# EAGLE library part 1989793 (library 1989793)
PCB terminal block, nominal current: 2 A, rated voltage (III/2): 250 V, nominal cross section: 0.5 mm, number of potentials: 7, number of rows: 1, number of positions per row: 7, product range: PTSA 0,5, pitch: 2.5 mm, connection method: Push-in spring connection, mounting: Wave soldering, conductor/PCB connection direction: 45 , color: green, Pin layout: Linear pinning, Solder pin [P]: 3.6 mm, number of solder pins per potential: 1, type of packaging: packed in cardboard. Soldering legs in front area, on Source: Datasheet
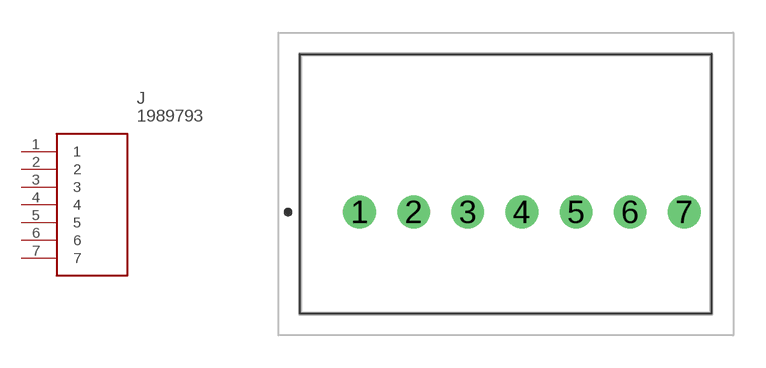
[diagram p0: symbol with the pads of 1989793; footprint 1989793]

Designator prefix J

## 1989793 (Description: PCB terminal block, nominal current: 2 A, rated voltage (III/2): 250 V, nominal cross section: 0.5 mm, number of potentials: 7, number of rows: 1, number of positions per row: 7, product range: PTSA 0,5, pitch: 2.5 mm, connection method: Push-in spring connection, mounting: Wave soldering, conductor/PCB connection direction: 45 , color: green, Pin layout: Linear pinning, Solder pin [P]: 3.6 mm, number of solder pins per potential: 1, type of packaging: packed in cardboard. Soldering legs in front area, on; Height: 13.1mm; Manufacturer_Name: Phoenix Contact; Manufacturer_Part_Number: 1989793; Mouser_Part_Number: 651-1989793; Mouser_Price-Stock: https://www.mouser.co.uk/ProductDetail/Phoenix-Contact/1989793?qs=sps7W%2FwBcGEvpTwR%2FpoOBQ%3D%3D)  [1989793]
1  1
2  2
3  3
4  4
5  5
6  6
7  7

## Footprint 1989793 (pad centres in mm)
1989793-2
drill 1 pad 1.5: 1 0,0; 2 2.5,0; 3 5,0; 4 7.5,0; 5 10,0; 6 12.5,0; 7 15,0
